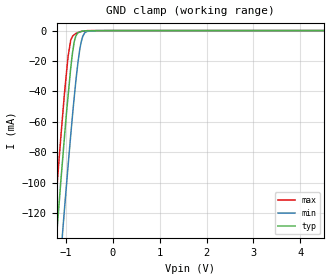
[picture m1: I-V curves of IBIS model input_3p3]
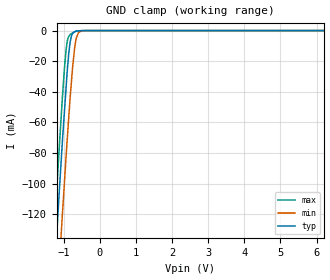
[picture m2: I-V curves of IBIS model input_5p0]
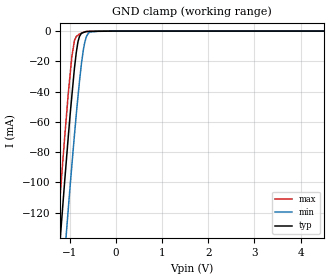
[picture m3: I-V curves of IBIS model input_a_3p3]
|Texas Instruments Incorporated
| High- or Low-Side Measurement,Bidirectional CURRENT/POWER MONITOR
| with 1.8V I2C Interface
| Marketing part#   Digital Voltage Range   Package-type   #pins
| INA231YFF   2.7V  - 5.5V   WCSP   12
[IBIS Ver]   3.2
[File name]   ina231.ibs
[File Rev]   1.0
[Date]   11/29/2012
[Source]
| Texas Instruments Incorporated.
| Analog-eLab Design Center, HPA
| 12500 TI Blvd
| Dallas, TX -75243
| e-mail: elab_scm_ibis@list.ti.com
[Notes]   Revision History:
| Rev 1.0: 11/29/2012
| - Initial version of the model
| - Model generated from simulations in TISPICE
| - Model matched to SPICE simulation
| - C_comp although listed in numerical order of value are
|   obtained from varying PVT conditions. For PVT conditions for
|   each specific value refer the buffer description under
|   respective [Model]. IBIS model user is responsible for using
|   appropriate C_comp to simulate for Signal Integrity.
| - Model names with a trailing _3p3 contains the model for
|   3.3V [3.0V and 3.6V]. Model names with a trailing _5p0 contains
|   the model for 5.0V [4.5V and 5.5V].
[Disclaimer]
| This model is designed as an aid for customers of Texas Instruments.
| TI and its licensors and suppliers make no warranties, either expressed
| or implied, with respect to this  model, including the warranties of
| merchantability or fitness for a particular purpose. The model is
| provided solely on an "as is" basis. The entire risk as to its quality
| and performance is with the customer.
[Copyright]
(C) Copyright 2012 Texas Instruments Incorporated.All rights reserved.
|   INA231
[Component]   INA231
[Manufacturer]   TI
[Package]   |WCSP-12
|   typ   min   max
R_pkg   0.00500   0.00500   0.00500
L_pkg   0.20000nH   0.20000nH   0.20000nH
C_pkg   0.60000pF   0.60000pF   0.60000pF
[Pin]  signal_name   model_name   R_pin   L_pin   C_pin
A1   IN+   term   0.00500   0.20000nH  0.60000pF
A2   IN-   term   0.00500   0.20000nH  0.60000pF
A3   BUS   term   0.00500   0.20000nH  0.60000pF
B1   A1   input   0.00500   0.20000nH  0.60000pF
B2   NC   NC   0.00500   0.20000nH  0.60000pF
B3   GND   GND   0.00500   0.20000nH  0.60000pF
C1   A0   input_a   0.00500   0.20000nH  0.60000pF
C2   NC   NC   0.00500   0.20000nH  0.60000pF
C3   VS   POWER   0.00500   0.20000nH  0.60000pF
D1   ALERT   alert   0.00500   0.20000nH  0.60000pF
D2   SDA   sda   0.00500   0.20000nH  0.60000pF
D3   SCL   scl   0.00500   0.20000nH  0.60000pF
|   Model Selectors
[Model Selector] input
input_3p3  3.3V digital input
input_5p0  5.0V digital input
[Model Selector] input_a
input_a_3p3  3.3V digital input
input_a_5p0  5.0V digital input
[Model Selector] alert
alert_3p3  3.3V digital open-drain
alert_5p0  5.0V digital open-drain
[Model Selector] sda
sda_3p3  3.3V digital I/0_open-drain
sda_5p0  5.0V digital I/0_open-drain
[Model Selector] scl
scl_3p3  3.3V digital input
scl_5p0  5.0V digital input
[Model Selector] term
term_3-3V  3.3V nominal termination
term_5-0V  5.0V nominal termination
[Model] term_3-3V
Model_type Terminator
C_comp   1.0e-20F  1.0e-20F  1.0e-20F
|   typ   min   max
[Voltage Range]   3.3V   3.0V   3.6V
[POWER Clamp Reference]   3.3V   3.0V   3.6V
[GND Clamp Reference]   0V   0V   0V
|Ambient Temperature   25   150   -65
|Junction Temperature
[Temperature Range]   27   125   -40
[Model] term_5-0V
Model_type Terminator
C_comp   1.0e-20F  1.0e-20F  1.0e-20F
|   typ   min   max
[Voltage Range]   5.0V   4.5V   5.5V
[POWER Clamp Reference]   5.0V   4.5V   5.5V
[GND Clamp Reference]   0V   0V   0V
|Ambient Temperature   25   150   -65
|Junction Temperature
[Temperature Range]   27   125   -40
| Models and submodels in the file (12): input_3p3 (Input), input_5p0 (Input), input_a_3p3 (Input), input_a_5p0 (Input), alert_3p3 (Open_drain), alert_5p0 (Open_drain), sda_3p3 (I/O_open_drain), sda_5p0 (I/O_open_drain), scl_3p3 (Input), scl_5p0 (Input), term_3-3V (Terminator), term_5-0V (Terminator)
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|   input_3p3 Model
[Model]   input_3p3
Model_type   Input
Vinl = 0.4
Vinh = 1.4
|   typ   min   max
|   (nom PVT)   (fast PVT)   (slow PVT)
|C_comp from frequency sweep method (F=100KHz)
|Average
|C_comp   1.183e-12   9.321e-13   1.483e-12
|C_comp from LC tank measurement(L=1nH)
|Average
|Resonant Frequency(Hz)   8.890e+09   9.410e+09   8.220e+09
C_comp   3.208e-13   2.863e-13   3.753e-13
| Where nom  PVT is Nominal Process, 3.3V, 27C
|   Fast PVT is Strong Process,  3.6V, -40C
|   Slow PVT is Weak Process,   3V, 125C
[Voltage Range]   3.3   3   3.6
|Ambient Temperature   25   150   -65
|Junction Temperature
[Temperature Range]   27   125   -40
[Power Clamp Reference]   3.3   3   3.6
[GND Clamp Reference]   0   0   0
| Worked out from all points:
|   GND clamp passes 1 mA (typ) near -0.71 V on its own axis
[GND Clamp]
|   Voltage   I(typ)   I(min)   I(max)
-3.3V     -1.016A    -1.05A     -997.6mA
-1.277V   -166.1mA   -214.2mA   -137.8mA
-1.161V   -120.1mA   -167.7mA   -90.78mA
-1.105V   -98.2mA    -146.4mA   -69.15mA
-1.033V   -70.85mA   -118.6mA   -42.29mA
-954mV    -43.22mA   -89.09mA   -17.09mA
-896.4mV  -24.4mA    -68.52mA   -6.187mA
-821.7mV  -7.312mA   -43.72mA   -2.71mA
-784.8mV  -3.378mA   -32.33mA   -1.848mA
-675mV    -619.7uA   -7.613mA   -555uA
-552mV    -208.7uA   -547.9uA   -75.11uA
6.6V      0A         0A         0A
[POWER Clamp]
|   Voltage   I(typ)   I(min)   I(max)
-3.3V     0A         0A         0A
-3.298V   0A         0A         0A
6.6V      0A         0A         0A
|   input_5p0 Model
[Model]   input_5p0
Model_type   Input
Vinl = 0.4
Vinh = 1.4
|   typ   min   max
|   (nom PVT)   (fast PVT)   (slow PVT)
|C_comp from frequency sweep method (F=100KHz)
|Average
|C_comp   1.066e-12   8.534e-13   1.316e-12
|C_comp from LC tank measurement(L=1nH)
|Average
|Resonant Frequency(Hz)   9.160e+09   9.570e+09   8.540e+09
C_comp   3.022e-13   2.769e-13   3.477e-13
| Where nom  PVT is Nominal Process, 5V, 27C
|   Fast PVT is Strong Process,  5.5V, -40C
|   Slow PVT is Weak Process,   4.5V, 125C
[Voltage Range]   5   4.5   5.5
|Ambient Temperature   25   150   -65
|Junction Temperature
[Temperature Range]   27   125   -40
[Power Clamp Reference]   5   4.5   5.5
[GND Clamp Reference]   0   0   0
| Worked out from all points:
|   GND clamp passes 1 mA (typ) near -0.72 V on its own axis
[GND Clamp]
|   Voltage   I(typ)   I(min)   I(max)
-5V       -1.739A    -1.766A    -1.726A
-1.368V   -203mA     -249.8mA   -174.9mA
-1.188V   -130.8mA   -178.2mA   -101.4mA
-1.122V   -104.7mA   -152.7mA   -75.46mA
-1.045V   -75.21mA   -123mA     -46.51mA
-940.5mV  -39.07mA   -84.19mA   -13.74mA
-902mV    -26.01mA   -70.49mA   -6.83mA
-820mV    -7.059mA   -43mA      -2.518mA
-670mV    -392.4uA   -6.945mA   -526.6uA
-589.5mV  -215.7uA   -1.247mA   -133uA
-373.5mV  -1.387uA   -6.98uA    -8.044uA
10V       0A         0A         0A
[POWER Clamp]
|   Voltage   I(typ)   I(min)   I(max)
-5V       0A         0A         0A
-5V       0A         0A         0A
10V       0A         0A         0A
|   input_a_3p3 Model
[Model]   input_a_3p3
Model_type   Input
Vinl = 0.4
Vinh = 1.4
|   typ   min   max
|   (nom PVT)   (fast PVT)   (slow PVT)
|C_comp from frequency sweep method (F=100KHz)
|Average
|C_comp   1.237e-12   9.668e-13   1.559e-12
|C_comp from LC tank measurement(L=1nH)
|Average
|Resonant Frequency(Hz)   8.880e+09   9.410e+09   8.220e+09
C_comp   3.215e-13   2.863e-13   3.753e-13
| Where nom  PVT is Nominal Process, 3.3V, 27C
|   Fast PVT is Strong Process,  3.6V, -40C
|   Slow PVT is Weak Process,   3V, 125C
[Voltage Range]   3.3   3   3.6
|Ambient Temperature   25   150   -65
|Junction Temperature
[Temperature Range]   27   125   -40
[Power Clamp Reference]   3.3   3   3.6
[GND Clamp Reference]   0   0   0
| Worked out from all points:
|   GND clamp passes 1 mA (typ) near -0.71 V on its own axis
[GND Clamp]
|   Voltage   I(typ)   I(min)   I(max)
-3.3V     -1.016A    -1.05A     -997.6mA
-1.277V   -166.1mA   -214.2mA   -137.8mA
-1.161V   -120.1mA   -167.7mA   -90.78mA
-1.105V   -98.2mA    -146.4mA   -69.15mA
-1.033V   -70.86mA   -118.6mA   -42.29mA
-954mV    -43.22mA   -89.09mA   -17.09mA
-896.4mV  -24.4mA    -68.53mA   -6.187mA
-821.7mV  -7.314mA   -43.72mA   -2.71mA
-784.8mV  -3.38mA    -32.33mA   -1.848mA
-675mV    -620.5uA   -7.616mA   -555uA
-552mV    -209.1uA   -552.7uA   -75.11uA
6.6V      0A         0A         0A
[POWER Clamp]
|   Voltage   I(typ)   I(min)   I(max)
-3.3V     0A         0A         0A
-3.298V   0A         0A         0A
6.6V      0A         0A         0A
